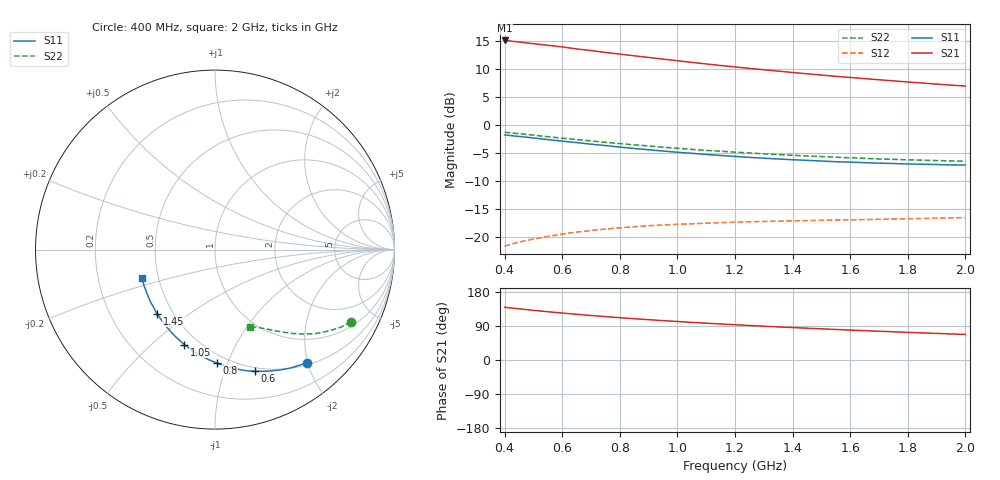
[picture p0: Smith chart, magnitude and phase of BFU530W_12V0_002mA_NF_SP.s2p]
! Filename:  P:\Prog\Test\Noise\ATS_data\Testdata_Net\06 Compressed Noise after Statistics\BFU530W_APM2013_09_A05_12p0V_002mA_NF_CM01_D.sf
! Date/Time: Tue 26/Mar/2013 18:06:02
! BFU530W_APM2013_09_A05_12p0V_1to25mA_NF_CM01_Bias2_R.sf
! Noise Parameter Data File
! BFU530W_APM2013_09_A05_12p0V_1to25mA_NF_CM01
! Date/time: Thu Mar 21 22:54:15 2013
! VAR V_out= 12.000000
! VAR I_out= 2.000000
! VAR V_in= 0.790800
! VAR I_in= 0.015695
! Device data file deembeded for feedlines and parallel
! Original file: \06 Compressed Noise after Statistics\BFU530W_APM2013_09_A05_12p0V_002mA_NF_CM01_R.sf
! Feed-files: PR019V01_070313_Feed1.s2p, PR019V01_070313_Feed2.s2p
! Parallel-file: PR019V01_070313_Par.s2p
# MHz S MA R 50
!  Freq-MHz  S11-mag  S11-arg  S21-mag  S21-arg  S12-mag  S12-arg  S22-mag  S22-arg
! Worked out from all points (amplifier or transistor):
!   37 points, 400 MHz to 2 GHz, reference 50 ohm
!   highest |S21| = 15.1 dB at 400 MHz (marker M1)
!   |S21| within 3 dB of that: start of sweep to 894.3 MHz
!   unconditionally stable (mu >= 1): nowhere
!   at 500 MHz: K = 0.28, MSG = 17.4 dB, |S12| = -20.4 dB
!   at 1.1 GHz: K = 0.57, MSG = 14.2 dB, |S12| = -17.6 dB
!   at 2 GHz: K = 0.93, MSG = 11.7 dB, |S12| = -16.6 dB
!   lowest NFmin = 0.53 dB at 420 MHz
!   S11 on the Smith chart (normalised r, x): 400 MHz: 0.54, -1.99; 600 MHz: 0.46, -1.28; 800 MHz: 0.43, -0.91; 1.05 GHz: 0.42, -0.64; 1.45 GHz: 0.41, -0.38; 2 GHz: 0.40, -0.16
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400  0.8121 -50.8  5.658 139.2  0.08248 60.7  0.8574 -28.0
420  0.8015 -53.1  5.598 137.4  0.08543 59.6  0.8478 -29.1
440  0.7916 -55.3  5.521 135.8  0.08819 58.5  0.838 -30.1
500  0.7617 -61.8  5.3 131.1  0.09557 55.6  0.8077 -33.0
550  0.7373 -66.8  5.126 127.4  0.1009 53.5  0.783 -35.2
600  0.7141 -71.8  4.954 123.9  0.1058 51.5  0.7594 -37.2
650  0.6935 -76.2  4.752 120.7  0.1102 49.7  0.7389 -39.0
700  0.6707 -80.9  4.602 117.4  0.1138 48.1  0.7171 -40.9
750  0.6521 -85.0  4.421 114.5  0.1173 46.6  0.6976 -42.3
800  0.632 -89.2  4.276 111.7  0.1203 45.4  0.6794 -43.8
850  0.6141 -93.3  4.128 108.9  0.123 44.2  0.6617 -45.2
950  0.5827 -100.8  3.858 103.9  0.1273 42.3  0.6303 -47.7
1050  0.5562 -107.8  3.605 99.3  0.1307 40.9  0.6027 -49.9
1150  0.532 -114.6  3.383 95.0  0.1339 39.7  0.5807 -51.8
1200  0.5217 -117.6  3.285 93.0  0.1349 39.4  0.5696 -52.9
1300  0.5031 -123.7  3.099 89.2  0.137 38.8  0.5506 -54.6
1450  0.4816 -132.2  2.852 83.9  0.1395 38.5  0.5267 -57.1
1500  0.4747 -134.9  2.778 82.2  0.1404 38.5  0.52 -58.0
1600  0.4641 -140.1  2.644 79.0  0.1417 38.8  0.5075 -59.6
1750  0.451 -147.4  2.466 74.5  0.1442 39.6  0.4915 -61.8
1850  0.4445 -152.1  2.358 71.5  0.1457 40.2  0.4833 -63.3
2000  0.4375 -158.8  2.216 67.5  0.1486 41.6  0.4725 -65.7
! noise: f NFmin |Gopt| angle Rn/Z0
400  0.5795  0.4507  24.97  0.1865
460  0.5555  0.4532  29.76  0.1925
600  0.5863  0.4472  36.2  0.2002
800  0.6392  0.4524  50.46  0.1727
1000  0.702  0.465  60.59  0.1772
1200  0.7564  0.4505  76.05  0.1563
1400  0.7815  0.4382  89.06  0.134
1600  0.7514  0.4331  104.2  0.107
1800  0.9114  0.4091  115.4  0.1028
2000  0.955  0.3833  127.5  0.1001
